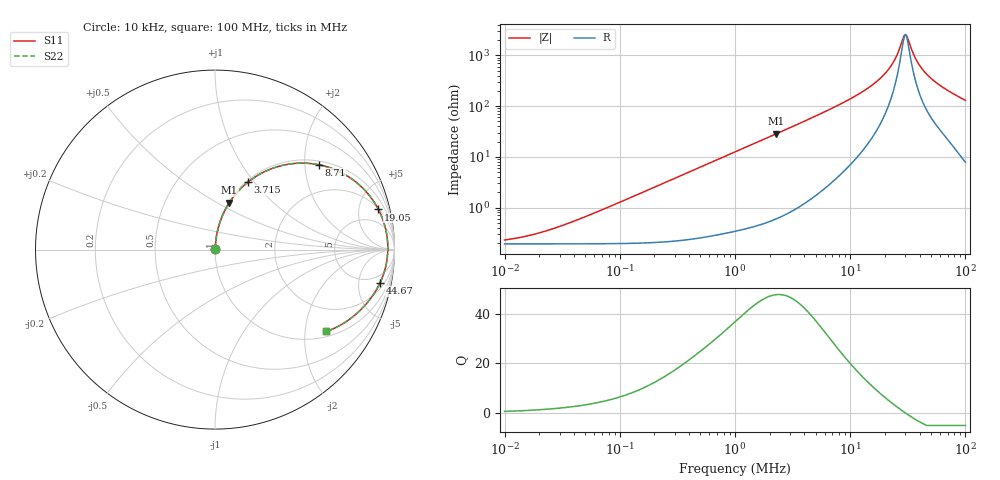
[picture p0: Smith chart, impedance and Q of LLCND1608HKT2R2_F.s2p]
! LLCND1608HKT2R2_F  S-PARAMETER MODEL  ( Standard Model )
! Model Generated by TAIYO YUDEN Corporation (http://www.ty-top.com)
! Version 1.0
! TAIYO YUDEN Control No. 220701
! Copyright(c) 2022 TAIYO YUDEN CO.,LTD. All Rights Reserved.
! Product Description (link to TY-COMPAS)
! https://ds.yuden.co.jp/TYCOMPAS/or/detail?pn=LLCND1608HKT2R2MF&u=M
! Products Name : Inductors
! Characteristics :
!  Inductance : 2.2 [uH] , SRF(min) : - [Hz] , DC Resistance(max) : 250 [mOhm]
!  Rated Current : Saturation  1.3 [A] (dL = 30 [%]), Temp Rise  1.4 [A] (dT = 40 [degC])
!  Case Size : 1.6 x 0.8 / 0.063 x 0.031 [mm/inch] , Thickness : 0.8 / 0.031 [mm/inch]
!  (Conditions: Temperature = 25 [degC] , DC Bias Current = 0 [A])
! External Node Assignments :
!  1  o---GGG---o  2
! GND o---------o GND
! Frequency Range : 10kHz  -  100MHz  [ 402 STEP ]
# MHz S RI R 50
! Freq[MHz].  S11 Real  S11 Imag  S21 Real  S21 Imag  S12 Real  S12 Imag  S22 Real  S22 Imag
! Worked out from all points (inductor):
!   401 points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, 10 kHz to 100 MHz, reference 50 ohm
!   read as one part in series: L = 2 uH near 46.77 kHz
!   highest Q = 47.6 at 2.291 MHz (marker M1), where L = 1.98 uH
!   self-resonance near 30.2 MHz
!   S11 on the Smith chart (normalised r, x): 10 kHz: 1.00, +0.00; 3.715 MHz: 1.02, +0.93; 8.71 MHz: 1.10, +2.35; 19.05 MHz: 2.08, +7.70; 44.67 MHz: 2.92, -9.03; 100 MHz: 1.16, -2.59
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0.01  0.00191 0.00125  0.9981 -0.00125  0.9981 -0.00125  0.00191 0.00125
0.020417  0.00192 0.00256  0.9981 -0.00256  0.9981 -0.00256  0.00192 0.00256
0.046774  0.00195 0.00586  0.998 -0.00586  0.998 -0.00586  0.00195 0.00586
0.218776  0.00281 0.0274  0.9972 -0.0274  0.9972 -0.0274  0.00281 0.0274
1  0.0185 0.1219  0.9815 -0.1219  0.9815 -0.1219  0.0185 0.1219
2.290868  0.0801 0.2612  0.9199 -0.2612  0.9199 -0.2612  0.0801 0.2612
3.715352  0.1848 0.3768  0.8152 -0.3768  0.8152 -0.3768  0.1848 0.3768
4.677351  0.2658 0.429  0.7342 -0.429  0.7342 -0.429  0.2658 0.429
6.456542  0.415 0.4767  0.585 -0.4767  0.585 -0.4767  0.415 0.4767
8.709636  0.5769 0.473  0.4231 -0.473  0.4231 -0.473  0.5769 0.473
13.48963  0.7955 0.368  0.2045 -0.368  0.2045 -0.368  0.7955 0.368
19.05461  0.9104 0.2239  0.0896 -0.2239  0.0896 -0.2239  0.9104 0.2239
21.87762  0.9382 0.1585  0.0618 -0.1585  0.0618 -0.1585  0.9382 0.1585
25.11886  0.9556 0.091  0.0444 -0.091  0.0444 -0.091  0.9556 0.091
28.84032  0.9627 0.0227  0.0373 -0.0227  0.0373 -0.0227  0.9627 0.0227
30.19952  0.9629 -2.67e-05  0.0371 2.67e-05  0.0371 2.67e-05  0.9629 -2.67e-05
31.62278  0.9618 -0.0227  0.0382 0.0227  0.0382 0.0227  0.9618 -0.0227
35.48134  0.9544 -0.0789  0.0456 0.0789  0.0456 0.0789  0.9544 -0.0789
38.01894  0.9467 -0.112  0.0533 0.112  0.0533 0.112  0.9467 -0.112
44.66836  0.9192 -0.1863  0.0808 0.1863  0.0808 0.1863  0.9192 -0.1863
61.6595  0.8297 -0.3168  0.1703 0.3168  0.1703 0.3168  0.8297 -0.3168
100  0.6204 -0.4559  0.3796 0.4559  0.3796 0.4559  0.6204 -0.4559
